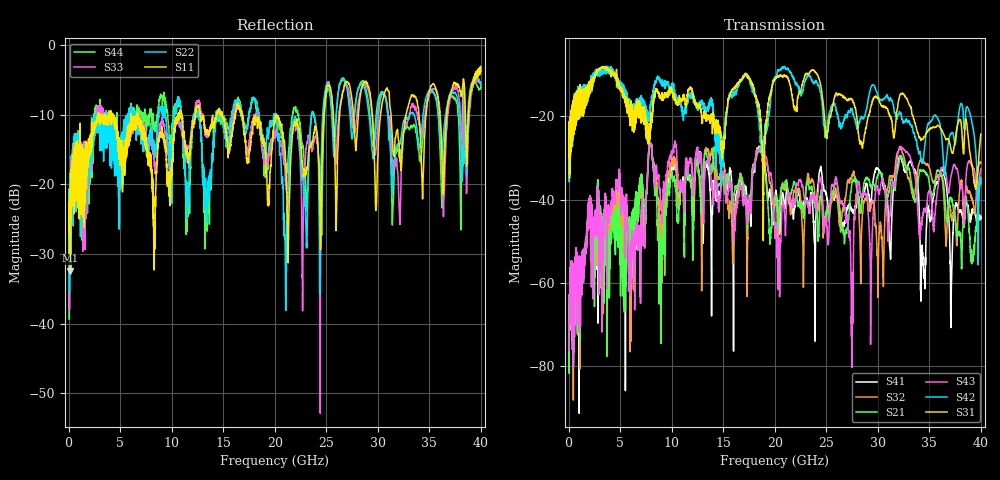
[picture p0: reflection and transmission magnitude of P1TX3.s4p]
!Agilent Technologies,N5245A,MY49151084,A.09.20.08
!Agilent N5245A: A.09.20.08
!Date: Thursday, March 01, 2012 11:59:40
!Correction: S11(Full 4 Port(1,2,3,4))
!S12(Full 4 Port(1,2,3,4))
!S13(Full 4 Port(1,2,3,4))
!S14(Full 4 Port(1,2,3,4))
!S21(Full 4 Port(1,2,3,4))
!S22(Full 4 Port(1,2,3,4))
!S23(Full 4 Port(1,2,3,4))
!S24(Full 4 Port(1,2,3,4))
!S31(Full 4 Port(1,2,3,4))
!S32(Full 4 Port(1,2,3,4))
!S33(Full 4 Port(1,2,3,4))
!S34(Full 4 Port(1,2,3,4))
!S41(Full 4 Port(1,2,3,4))
!S42(Full 4 Port(1,2,3,4))
!S43(Full 4 Port(1,2,3,4))
!S44(Full 4 Port(1,2,3,4))
!S4P File: Measurements: <S11,S12,S13,S14>,
!<S21,S22,S23,S24>,
!<S31,S32,S33,S34>,
!<S41,S42,S43,S44>:
# Hz S  dB  R 50
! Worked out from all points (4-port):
!   3996 points, 50 MHz to 40 GHz, reference 50 ohm
!   strongest paths, dB at 50 MHz, 10.04 GHz, 20.03 GHz, 30.02 GHz, 40 GHz:
!     S31: -25.2, -14.0, -11.1, -15.8, -24.3
!     S42: -24.6, -12.8, -10.7, -15.1, -36.2
!     S43: -72.8, -28.6, -48.9, -37.7, -32.6
!     S21: -63.6, -34.2, -39.7, -34.2, -34.8
!     S32: -73.3, -30.8, -40.4, -61.4, -31.3
!     S41: -62.9, -31.9, -39.9, -32.7, -44.5
!   lowest |S11| = -32.4 dB at 180 MHz (marker M1), VSWR 1.05, Z = 52.4 + j0.27 ohm
!   |S11| at or under -10 dB: 6.7 GHz to 10.63 GHz (3.927 GHz wide, 45.3 % of centre); 16.83 GHz to 20.17 GHz (3.343 GHz wide, 18.1 % of centre); 20.18 GHz to 24.76 GHz (4.582 GHz wide, 20.4 % of centre)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
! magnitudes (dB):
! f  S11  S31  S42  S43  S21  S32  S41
! 50 MHz  -24.8  -25.2  -24.6  -72.8  -63.6  -73.3  -62.9
! 180 MHz  -32.4  -29.4  -27.0  -61.7  -60.4  -60.8  -61.6
! 7.94 GHz  -16.2  -21.7  -17.0  -26.6  -26.4  -26.7  -26.6
! 8.91 GHz  -12.5  -15.4  -11.4  -40.8  -51.3  -44.7  -50.6
! 18.84 GHz  -14.1  -33.7  -28.1  -27.6  -28.4  -27.6  -27.5
! 27.46 GHz  -7.4  -16.0  -18.2  -69.8  -36.6  -34.7  -42.4
! 40 GHz  -3.8  -24.3  -36.2  -32.6  -34.8  -31.3  -44.5
